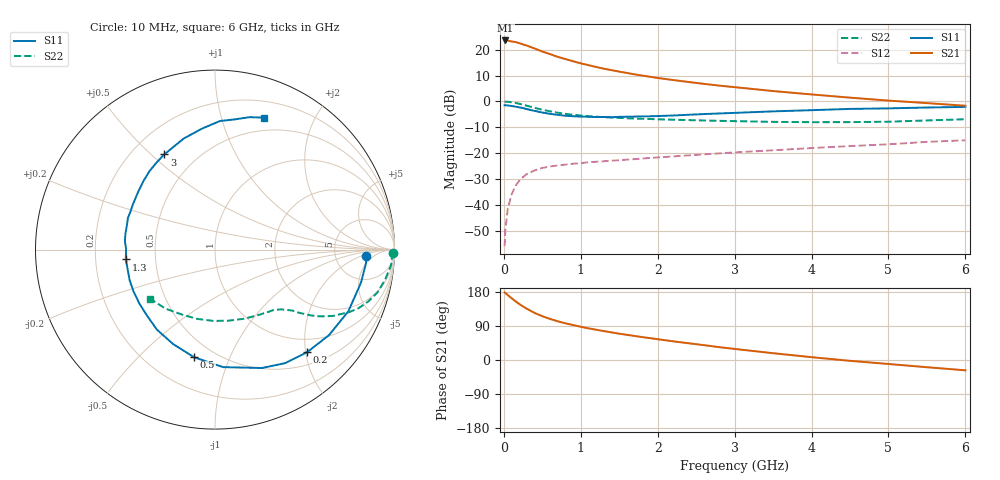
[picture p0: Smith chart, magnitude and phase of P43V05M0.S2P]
! SIEMENS Small Signal Semiconductors
! BFP182
! Si NPN RF Bipolar Junction Transistor in SOT143
! VCE = 3 V  IC = 5 mA
! Common Emitter S-Parameters:  March  1996
# GHz  S  MA  R  50
!  f  S11  S21  S12  S22
! GHz  MAG  ANG  MAG  ANG  MAG  ANG  MAG  ANG
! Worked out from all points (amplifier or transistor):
!   36 points, 10 MHz to 6 GHz, reference 50 ohm
!   highest |S21| = 23.6 dB at 20 MHz (marker M1)
!   |S21| within 3 dB of that: start of sweep to 390.8 MHz
!   unconditionally stable (mu >= 1): 1.6 GHz to 5.499 GHz
!   at 250 MHz: K = 0.21, MSG = 25.6 dB, |S12| = -29.2 dB
!   at 1.4 GHz: K = 0.93, MSG = 17.5 dB, |S12| = -22.9 dB
!   at 6 GHz: K = 0.94, MSG = 6.7 dB, |S12| = -15.0 dB
!   lowest NFmin = 1.20 dB at 450 MHz
!   S11 on the Smith chart (normalised r, x): 10 MHz: 11, -3; 200 MHz: 0.72, -2.02; 500 MHz: 0.39, -0.75; 1.3 GHz: 0.33, -0.05; 3 GHz: 0.33, +0.55; 6 GHz: 0.36, +1.37
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0.01  0.8438 -2.4  14.83 178.4  0.0016 76.6  0.9902 -1.0
0.02  0.8447 -5.2  15.05 177.0  0.0033 89.5  0.9873 -2.0
0.05  0.834 -12.7  14.92 171.4  0.0082 86.1  0.985 -5.1
0.1  0.8187 -24.8  14.41 163.2  0.0159 77.2  0.9627 -10.0
0.15  0.7941 -36.9  14.05 155.1  0.0233 70.5  0.9365 -14.7
0.2  0.7681 -48.2  13.38 147.8  0.0293 65.4  0.9016 -18.7
0.25  0.7431 -58.4  12.6 141.2  0.0347 60.6  0.8641 -22.2
0.3  0.7096 -68.4  11.98 135.2  0.0397 56.7  0.8246 -25.0
0.4  0.6563 -86.1  10.53 124.2  0.0465 50.0  0.7516 -29.5
0.5  0.6108 -101.0  9.196 115.6  0.0518 44.9  0.6924 -32.5
0.6  0.5757 -113.9  8.203 108.4  0.0555 41.2  0.6448 -34.6
0.7  0.5511 -125.9  7.268 102.2  0.0579 38.9  0.6058 -36.1
0.9  0.5178 -144.4  5.971 92.2  0.0626 35.8  0.5516 -38.1
1.1  0.5053 -160.3  5.017 83.5  0.0669 34.4  0.5197 -40.2
1.3  0.5 -173.7  4.289 76.3  0.0699 33.4  0.4967 -42.1
1.7  0.5094 164.5  3.334 63.4  0.0767 33.2  0.4656 -46.7
2.2  0.5345 143.6  2.588 49.3  0.0866 32.5  0.4439 -53.8
3  0.6007 118.1  1.886 29.2  0.1036 31.1  0.416 -68.3
3.5  0.6427 105.8  1.586 17.9  0.1138 29.1  0.4032 -79.1
4.5  0.7169 87.8  1.183 -2.2  0.1371 24.5  0.3981 -103.9
5.5  0.7624 75.4  0.928 -19.1  0.1654 19.1  0.429 -129.9
6  0.7841 69.7  0.825 -27.2  0.1776 14.9  0.453 -142.5
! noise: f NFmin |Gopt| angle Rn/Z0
0.45  1.2  0.27  37  0.3
0.9  1.3  0.25  75  0.23
1.8  1.9  0.21  145  0.2
